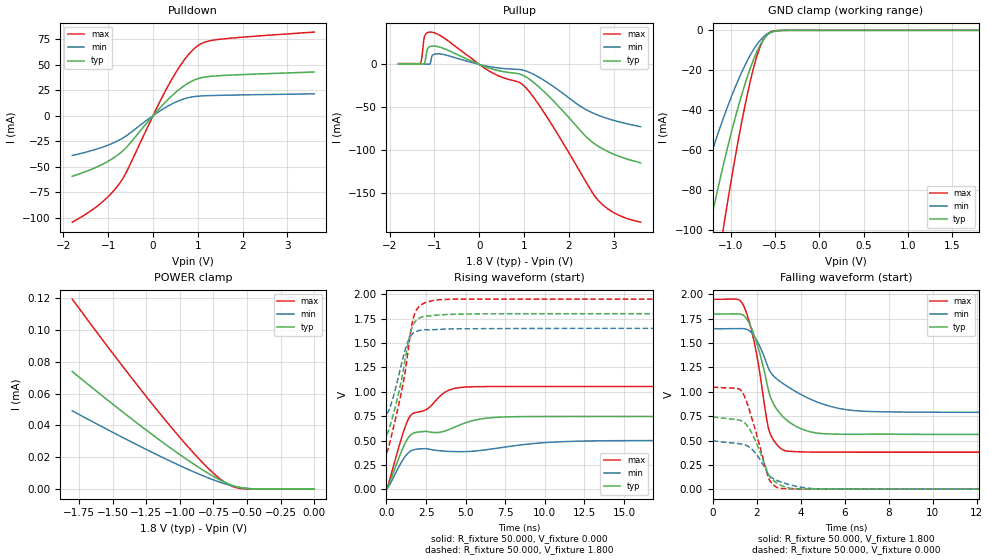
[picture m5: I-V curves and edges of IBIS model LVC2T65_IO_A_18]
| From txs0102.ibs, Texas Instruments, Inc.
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[Model]   LVC2T65_IO_A_18
Model_type  I/O
Vinl=0.15
Vinh=1.45
Enable   Active-High
Vref =   1.8V
Rref =   1000000
Cref =   15p
Vmeas =   0.9
| variable   typ   min   max
C_comp   5.39pF   4.65pF   5.79pF
| C_pullup   6.08pF   4.69pF   7.53pF
| C_pulldown   6.31pF   5.25pF   7.69pF
| C_tri-state   5.39pF   4.65pF   5.79pF
[Temperature Range]   40   100   -40
| Ambient temperature   25   85   -40
[Voltage range]   1.8   1.65   1.95
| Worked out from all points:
|   slope of the pulldown table from 0 to 0.27 V, typ, clamps not added: 20.7 ohm
|   slope of the pullup table from 0 to 0.27 V, typ, clamps not added: 53.6 ohm
|   GND clamp passes 1 mA (typ) near -0.54 V on its own axis
|   rising waveform, R_fixture 50.000, V_fixture 0.000: 20-80 % time 3.26ns typ, 1.23ns min, 2.32ns max; typ from 0.003 V to 0.745 V
|   falling waveform, R_fixture 50.000, V_fixture 1.800: 20-80 % time 1.02ns typ, 2.07ns min, 718ps max; typ from 1.8 V to 0.562 V
|   rising waveform, R_fixture 50.000, V_fixture 1.800: 20-80 % time 934ps typ, 834ps min, 1.03ns max; typ from 0.561 V to 1.8 V
|   falling waveform, R_fixture 50.000, V_fixture 0.000: 20-80 % time 807ps typ, 994ps min, 787ps max; typ from 0.745 V to 0.002 V
[GND Clamp]
| LVC2T65_IO_A_18
|   Voltage   I(typ)   I(min)   I(max)
-1.8V     -231.8mA   -156.9mA   -331.5mA
-1.45V    -145.7mA   -96.71mA   -212.6mA
-1.265V   -104.5mA   -68.67mA   -153.7mA
-1.22V    -95.02mA   -62.32mA   -139.9mA
-1.08V    -67.3mA    -43.9mA    -98.97mA
-1.06V    -63.57mA   -41.44mA   -93.4mA
-920mV    -39.42mA   -25.62mA   -56.87mA
-785mV    -19.97mA   -13.05mA   -27.02mA
-680mV    -8.524mA   -5.772mA   -9.919mA
-585mV    -2.39mA    -1.79mA    -1.977mA
-370mV    -14.85uA   -19.53uA   -2.704uA
1.8V      189.3pA    1.871nA    43.31pA
[POWER Clamp]
| LVC2T65_IO_A_18
|   Voltage   I(typ)   I(min)   I(max)
-1.8V     73.89uA    49.21uA    119.4uA
-1.4V     46.86uA    31.38uA    74.43uA
-1.1V     27.74uA    18.78uA    42.58uA
-975mV    20.24uA    13.85uA    30.1uA
-855mV    13.44uA    9.39uA     18.85uA
-770mV    9.017uA    6.485uA    11.6uA
-695mV    5.54uA     4.192uA    6.115uA
-620mV    2.727uA    2.293uA    2.164uA
-530mV    718.5nA    790.7nA    265.8nA
-395mV    37.08nA    77.03nA    3.477nA
0V        0A         0A         0A
[Pulldown]
| LVC2T65_IO_A_18
|   Voltage   I(typ)   I(min)   I(max)
-1.8V     -59.5mA    -39.09mA   -104.6mA
-1.2V     -49.37mA   -32.07mA   -87.36mA
-945mV    -43.37mA   -27.96mA   -77.09mA
-740mV    -37.1mA    -23.72mA   -66.24mA
-570mV    -30.1mA    -19.06mA   -53.51mA
50mV      2.359mA    1.439mA    4.301mA
390mV     18.08mA    10.68mA    33.19mA
710mV     29.69mA    16.68mA    55.27mA
955mV     35.51mA    18.87mA    67.04mA
1.155V    37.84mA    19.48mA    72.05mA
1.405V    38.98mA    19.83mA    74.44mA
3.6V      42.82mA    21.38mA    82mA
[Pullup]
| LVC2T65_IO_A_18
|   Voltage   I(typ)   I(min)   I(max)
-1.8V     493.8uA    242.7uA    970.1uA
-1.32V    482uA      237uA      1.134mA
-1.285V   481.3uA    236.1uA    6.641mA
-1.215V   2.168mA    234.4uA    33.49mA
-1.155V   18.02mA    233.1uA    36.99mA
-1.095V   20.83mA    656.5uA    37.66mA
-1.06V    21.3mA     9.086mA    37.54mA
215mV     -4.145mA   -2.416mA   -7.489mA
915mV     -11.38mA   -6.038mA   -21.43mA
1.355V    -27.19mA   -15.59mA   -48.7mA
2.655V    -95.2mA    -59.16mA   -158.3mA
3.6V      -114.6mA   -72.52mA   -183.7mA
[Ramp]
| LVC2T65_IO_A_18
| variable   typ   min   max
dV/dt_r   0.48/3.29E-09   0.32/1.25E-09   0.66/2.33E-09
dV/dt_f   0.73/1.02E-09   0.50/2.07E-09   0.94/7.19E-10
R_load = 50
[Rising Waveform]
R_fixture = 50.000
V_fixture = 0.000
V_fixture_min = 0.000
V_fixture_max = 0.000
C_fixture = 0.000
L_fixture = 0.000
|  time   V(typ)   V(min)   V(max)
0s        2.669mV    2.533mV    2.724mV
1.092ns   443.2mV    317mV      598.9mV
1.512ns   555.7mV    391.7mV    754.8mV
2.604ns   591.8mV    415.1mV    827.3mV
3.444ns   587.9mV    395.2mV    964.8mV
4.032ns   619.1mV    388.7mV    1.022V
5.712ns   714.6mV    395.4mV    1.053V
10.42ns   747mV      483.3mV    1.054V
16.97ns   747.1mV    500.5mV    1.054V
419.9ns   745.1mV    499.1mV    1.051V
[Falling Waveform]
R_fixture = 50.000
V_fixture = 1.800
V_fixture_min = 1.650
V_fixture_max = 1.950
C_fixture = 0.000
L_fixture = 0.000
|  time   V(typ)   V(min)   V(max)
0s        1.8V       1.65V      1.95V
1.344ns   1.79V      1.647V     1.908V
1.848ns   1.601V     1.581V     1.546V
2.436ns   1.115V     1.3V       739.6mV
2.604ns   957.7mV    1.208V     573.2mV
3.192ns   744mV      1.084V     404.3mV
4.284ns   599.1mV    940.2mV    383mV
6.3ns     564.3mV    810.4mV    381mV
10.75ns   563.3mV    790.2mV    381mV
419.9ns   561.8mV    776.2mV    380.3mV
[Rising Waveform]
R_fixture = 50.000
V_fixture = 1.800
V_fixture_min = 1.650
V_fixture_max = 1.950
C_fixture = 0.000
L_fixture = 0.000
|  time   V(typ)   V(min)   V(max)
0s        561.4mV    775.7mV    369.8mV
336ps     711.1mV    895.7mV    563.2mV
1.008ns   1.171V     1.323V     1.047V
1.176ns   1.325V     1.426V     1.198V
1.428ns   1.548V     1.543V     1.498V
1.596ns   1.651V     1.586V     1.68V
1.764ns   1.709V     1.609V     1.791V
2.352ns   1.772V     1.635V     1.906V
3.864ns   1.792V     1.643V     1.948V
419.9ns   1.8V       1.65V      1.95V
[Falling Waveform]
R_fixture = 50.000
V_fixture = 0.000
V_fixture_min = 0.000
V_fixture_max = 0.000
C_fixture = 0.000
L_fixture = 0.000
|  time   V(typ)   V(min)   V(max)
0s        744.8mV    498.7mV    1.05V
1.092ns   714mV      470.7mV    1.034V
1.344ns   698mV      463.2mV    997.3mV
1.848ns   543.2mV    395.8mV    674.7mV
2.52ns    155.9mV    155.9mV    120.3mV
2.604ns   124.8mV    132.8mV    84.59mV
3.024ns   51.47mV    82.24mV    12.12mV
3.864ns   6.513mV    28.57mV    3.732mV
8.484ns   2.482mV    2.199mV    2.615mV
419.9ns   2.384mV    2.058mV    2.611mV
